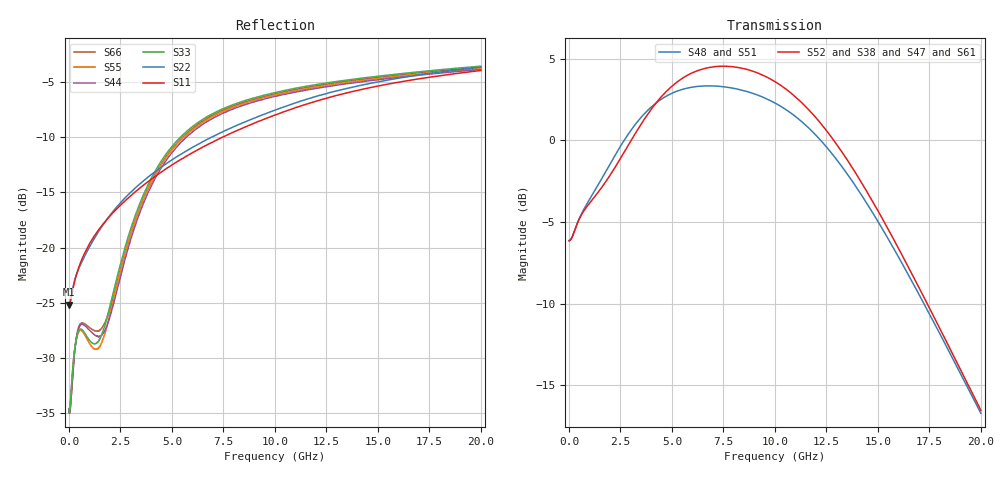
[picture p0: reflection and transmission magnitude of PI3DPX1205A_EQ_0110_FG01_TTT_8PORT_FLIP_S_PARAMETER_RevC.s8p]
! NPort=8 DATA=2000 NOISE=0 GROUPDELAY=0 COMPLEX_DATAFORMAT=POLAR
! NumOfBlock=1 NumOfParam=0
! .MODEL Smodel S TSTONEFILE=PI3DPX1205A_EQ_0110_FG01_TTT_8PORT_FLIP_S_PARAMETER_RevC.s8p TYPE=S
!  -- The above .MODEL line can be used for the S element in the netlist.
! The s parameter is extracted from the linear redriver, it is not bi-directional;
! only s(5,1)s(6,2)s(3,7)s(4,8) should be the insertion loss
!  Port definition:
!  Port1 = AIP
!  Port2 = AIN
!  Port3 = BOP
!  Port4 = BON
!  Port5 = AOP
!  Port6 = AON
!  Port7 = BIP
!  Port8 = BIN
# Hz S MA R  50
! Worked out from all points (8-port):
!   2000 points, 10 MHz to 20 GHz, reference 50 ohm
!   strongest paths, dB at 10 MHz, 5.01 GHz, 10.01 GHz, 15.01 GHz, 20 GHz:
!     S52: -6.1, 3.3, 3.6, -4.3, -16.5
!     S38: -6.1, 3.3, 3.6, -4.3, -16.5
!     S47: -6.1, 3.3, 3.6, -4.3, -16.5
!     S61: -6.1, 3.3, 3.6, -4.3, -16.5
!     S48: -6.1, 2.9, 2.3, -5.0, -16.7
!     S51: -6.1, 2.9, 2.3, -5.0, -16.7
!   lowest |S11| = -25.2 dB at 10 MHz (marker M1), VSWR 1.12, Z = 44.8 - j0.115 ohm
!   |S11| at or under -10 dB: start of sweep to 7.465 GHz
